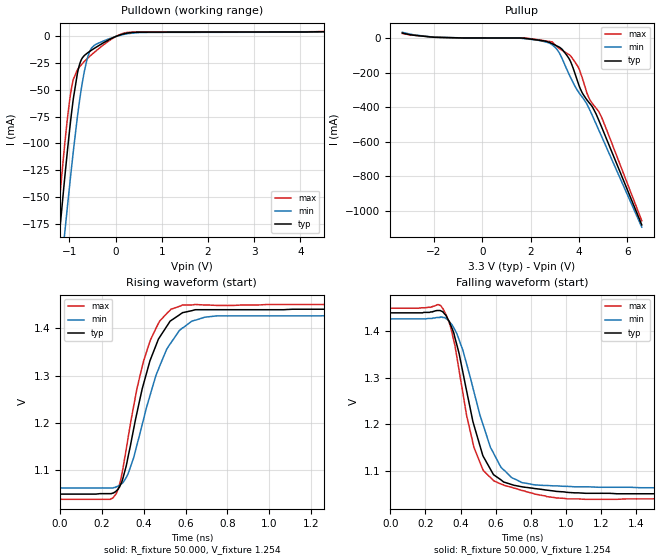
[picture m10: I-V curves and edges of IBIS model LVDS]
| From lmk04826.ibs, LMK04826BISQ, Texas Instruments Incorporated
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[Model]   LVDS
Model_type   Output
Polarity   Non-Inverting
Vmeas = 1.254
Vref = 1.254
Cref = 15pF
Rref = 50
|   typ   min   max
|   (fast PVT)   (nom PVT)   (slow PVT)
C_comp   2.419p   2.365p   2.604p
|C_comp (high state)   2.207p   1.674p   2.323p
|C_comp (low state)   2.419p   2.365p   2.604p
| Where   nom PVT is  Nominal Process, 3.3V, 27C
|   Fast PVT is Strong Process, 3.45V, -40C
|   Slow PVT is Weak Process, 3.15V, 125C
[Voltage Range]   3.3   3.15   3.45
[Temperature Range]   27   125   -40
[Pullup Reference]   3.3   3.15   3.45
[Pulldown Reference]   0   0   -0
[Power Clamp Reference]   3.3   3.15   3.45
[GND Clamp Reference]   0   0   0
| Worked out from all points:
|   slope of the pulldown table from 0 to 0.495 V, typ, clamps not added: 122 ohm
|   slope of the pullup table from 0 to 0.495 V, typ, clamps not added: 8.01 kohm
|   falling waveform, R_fixture 50.000, V_fixture 1.254: 20-80 % time 148ps typ, 173ps min, 138ps max; typ from 1.44 V to 1.05 V
|   rising waveform, R_fixture 50.000, V_fixture 1.254: 20-80 % time 132ps typ, 151ps min, 119ps max; typ from 1.05 V to 1.44 V
[Pulldown]
|   Voltage   I(typ)   I(min)   I(max)
-3.3V     -1.212A    -1.183A    -1.242A
-1.27V    -210.5mA   -257.4mA   -180.1mA
-1.231V   -191.8mA   -240mA     -160.8mA
-1.092V   -128.3mA   -180mA     -96.92mA
-993.3mV  -86.54mA   -138.5mA   -59.29mA
-914.1mV  -57.9mA    -106.9mA   -39.97mA
-795.3mV  -28.47mA   -64.69mA   -29.24mA
-676.5mV  -17.81mA   -32.66mA   -23.35mA
-518.1mV  -12.71mA   -10.69mA   -16.95mA
-270.6mV  -6.088mA   -4.327mA   -8.117mA
283.8mV   3.422mA    2.749mA    3.938mA
6.59V     5.723mA    5.795mA    5.697mA
[Pullup]
|   Voltage   I(typ)   I(min)   I(max)
-3.3V     28.69mA    32.84mA    26.16mA
-1.954V   4.023mA    4.845mA    4.182mA
2.224V    -10.47mA   -11.77mA   -8.431mA
2.818V    -28.07mA   -32.53mA   -20.83mA
3.204V    -54.46mA   -91mA      -62.46mA
3.62V     -128mA     -219.5mA   -99.52mA
3.977V    -265.8mA   -312.1mA   -171.7mA
4.135V    -317.9mA   -342.1mA   -231.9mA
4.402V    -371.6mA   -404.4mA   -344.8mA
4.699V    -438mA     -495.7mA   -405.3mA
4.947V    -519.8mA   -574.1mA   -463.4mA
6.59V     -1.08A     -1.093A    -1.057A
[Ramp]
R_load = 50
|   typ   min   max
dV/dt_r   0.226512/1.32224e-10   0.209748/1.5098e-10   0.239484/1.19685e-10
dV/dt_f   0.226806/1.48005e-10   0.210087/1.735e-10   0.239728/1.38322e-10
[Falling Waveform]
R_fixture = 50.000
V_fixture = 1.254
V_fixture_min = 1.254
V_fixture_max = 1.254
C_fixture = 0.000
|  time   V(typ)   V(min)   V(max)
0s        1.44V      1.427V     1.45V
299.9ps   1.442V     1.43V      1.449V
361ps     1.397V     1.408V     1.38V
433.6ps   1.273V     1.331V     1.22V
475.8ps   1.198V     1.27V      1.15V
529.6ps   1.13V      1.197V     1.1V
648ps     1.075V     1.101V     1.068V
749.8ps   1.065V     1.074V     1.057V
1.05ns    1.052V     1.065V     1.039V
3ns       1.05V      1.063V     1.039V
[Rising Waveform]
R_fixture = 50.000
V_fixture = 1.254
V_fixture_min = 1.254
V_fixture_max = 1.254
C_fixture = 0.000
|  time   V(typ)   V(min)   V(max)
0s        1.05V      1.063V     1.039V
266.7ps   1.056V     1.065V     1.05V
288.7ps   1.07V      1.07V      1.079V
324.9ps   1.129V     1.093V     1.169V
368ps     1.223V     1.155V     1.274V
429.2ps   1.331V     1.257V     1.372V
509.8ps   1.404V     1.356V     1.431V
586ps     1.433V     1.401V     1.449V
749.8ps   1.439V     1.426V     1.448V
3ns       1.44V      1.427V     1.45V
